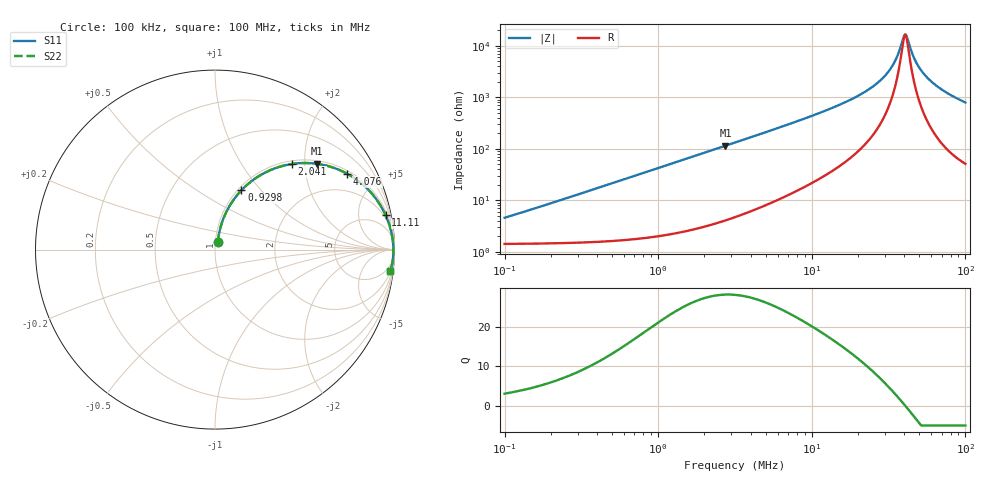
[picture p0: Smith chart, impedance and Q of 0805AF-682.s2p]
# MHz  S  MA  R  50
!Freq  MagS11  AngS11  MagS21  AngS21  MagS12  AngS12  MagS22  AngS22
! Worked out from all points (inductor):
!   801 points, 100 kHz to 100 MHz, reference 50 ohm
!   read as one part in series: L = 6.92 uH near 103.5 kHz
!   highest Q = 28.2 at 2.739 MHz (marker M1), where L = 6.68 uH
!   self-resonance near 40.26 MHz
!   S11 on the Smith chart (normalised r, x): 100 kHz: 1.03, +0.09; 929.8 kHz: 1.04, +0.79; 2.041 MHz: 1.06, +1.72; 4.076 MHz: 1.12, +3.42; 11.11 MHz: 1.52, +9.83; 100 MHz: 2, -16
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0.1  0.04522 69.5  0.9851 -2.5  0.9851 -2.5  0.04522 69.5
0.3183882  0.1344 76.0  0.9763 -7.7  0.9763 -7.7  0.1344 76.0
0.929779  0.3611 66.0  0.9149 -21.1  0.9149 -21.1  0.3611 66.0
1.004987  0.3856 64.6  0.9047 -22.7  0.9047 -22.7  0.3856 64.6
2.041456  0.64 48.2  0.7454 -39.8  0.7454 -39.8  0.64 48.2
2.738772  0.7416 40.1  0.6451 -47.8  0.6451 -47.8  0.7416 40.1
3.172224  0.7862 36.2  0.5907 -51.8  0.5907 -51.8  0.7862 36.2
4.075799  0.8499 29.8  0.4968 -58.1  0.4968 -58.1  0.8499 29.8
6.224864  0.9225 20.5  0.3503 -67.2  0.3503 -67.2  0.9225 20.5
10.01307  0.9646 12.7  0.2204 -74.4  0.2204 -74.4  0.9646 12.7
11.1073  0.9701 11.4  0.1971 -75.6  0.1971 -75.6  0.9701 11.4
21.98506  0.9896 4.5  0.0784 -80.2  0.0784 -80.2  0.9896 4.5
27.28745  0.9921 2.8  0.04946 -79.4  0.04946 -79.4  0.9921 2.8
31.88044  0.9932 1.7  0.03007 -76.2  0.03007 -76.2  0.9932 1.7
35.67128  0.9938 0.9  0.0168 -67.7  0.0168 -67.7  0.9938 0.9
39.56941  0.994 0.2  0.006727 -27.2  0.006727 -27.2  0.994 0.2
40.96125  0.9941 -0.1  0.006035 10.3  0.006035 10.3  0.9941 -0.1
42.03717  0.9941 -0.2  0.007263 35.3  0.007263 35.3  0.9941 -0.2
47.44399  0.994 -1.1  0.01981 71.8  0.01981 71.8  0.994 -1.1
55.4297  0.9934 -2.2  0.03873 79.1  0.03873 79.1  0.9934 -2.2
70.60542  0.9913 -4.0  0.0706 80.9  0.0706 80.9  0.9913 -4.0
100  0.9844 -7.1  0.1238 79.2  0.1238 79.2  0.9844 -7.1
